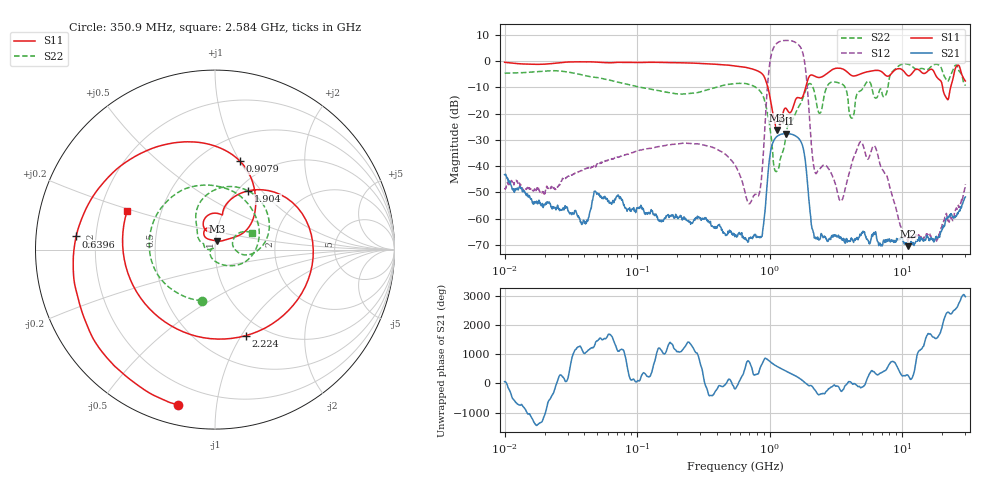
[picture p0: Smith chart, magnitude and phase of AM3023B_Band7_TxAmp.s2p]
# Hz S DB R 50.0
!freq dBS11 angS11 dBS21 angS21 dBS12 angS12 dBS22 angS22
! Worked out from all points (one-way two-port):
!   1601 points, 10 MHz to 30 GHz, reference 50 ohm
!   highest |S21| = -27.61 dB at 1.321 GHz (marker M1); lowest = -70.6 dB at 11.03 GHz (marker M2)
!   lowest |S11| = -26.2 dB at 1.137 GHz (marker M3), VSWR 1.10, Z = 50.8 + j4.9 ohm
!   |S11| at or under -10 dB: 970.2 MHz to 1.869 GHz (898.9 MHz wide, 63.3 % of centre); 20.2 GHz to 23.2 GHz (2.994 GHz wide, 13.8 % of centre)
!   |S22| runs from -42.1 to -0.9 dB; largest |S21 - S12| = 2.5
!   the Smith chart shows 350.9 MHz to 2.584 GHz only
!   S11 on the Smith chart (normalised r, x): 350.9 MHz: 0.09, -0.79; 639.6 MHz: 0.13, +0.05; 907.9 MHz: 0.75, +1.00; 1.904 GHz: 1.11, +0.85; 2.224 GHz: 0.81, -1.04; 2.584 GHz: 0.32, +0.19
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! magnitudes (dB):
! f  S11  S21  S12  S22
! 10 MHz  -0.4  -43.2  -48.8  -4.6
! 38.04 MHz  -0.2  -62.1  -41.7  -5.2
! 49.1 MHz  -0.3  -50.0  -39.9  -6.2
! 144.7 MHz  -0.4  -60.7  -32.6  -11.2
! 350.9 MHz  -1.0  -61.7  -32.5  -10.6
! 547.7 MHz  -1.8  -66.3  -39.6  -8.5
! 639.6 MHz  -2.2  -67.6  -48.3  -8.4
! 825.6 MHz  -3.9  -67.1  -51.2  -10.8
! 907.9 MHz  -5.8  -60.3  -30.5  -14.3
! 1.004 GHz  -13.5  -36.2  -0.6  -25.2
! 1.137 GHz  -26.2  -28.7  6.9  -41.9
! 1.321 GHz  -17.9  -27.6  7.9  -28.9
! 1.904 GHz  -8.5  -43.0  -7.3  -9.8
! 2.084 GHz  -5.2  -63.6  -34.2  -9.1
! 2.224 GHz  -5.9  -67.2  -42.7  -14.1
! 2.584 GHz  -5.4  -67.2  -39.6  -12.9
! 3.471 GHz  -2.8  -67.6  -53.3  -8.5
! 4.156 GHz  -5.4  -67.9  -39.1  -21.7
! 4.878 GHz  -4.8  -66.4  -30.7  -11.2
! 7.926 GHz  -5.6  -67.9  -46.3  -7.6
! 11.03 GHz  -5.5  -70.6  -68.5  -1.1
! 30 GHz  -7.5  -51.8  -46.9  -9.3
